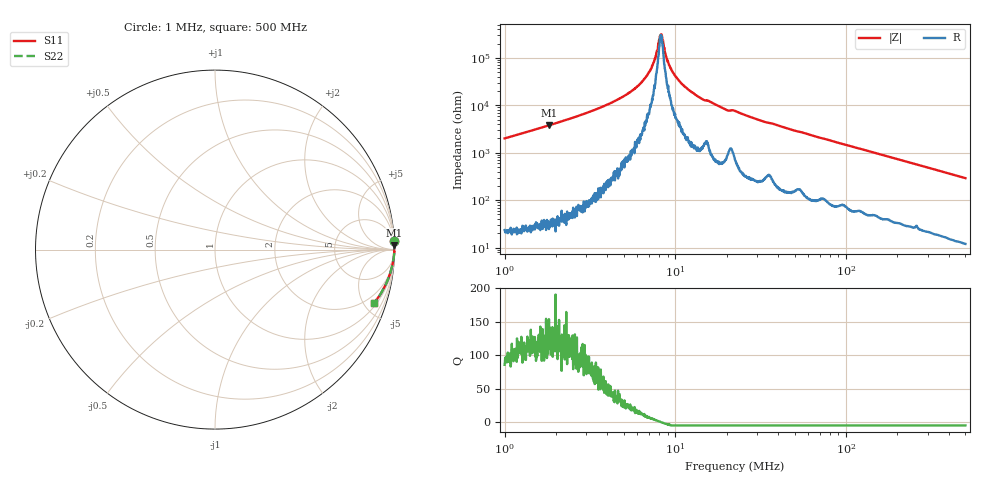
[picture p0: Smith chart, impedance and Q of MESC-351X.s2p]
!s-Parameter Generated by FASTRON Sdn. Bhd.
!FASTRON P/N : MESC-351X
!Keysight Technologies,E4991B,MY54100416,A.01.15
!Date: Fri Mar 27 11:36:06 2026
!Version  : Rev00 Fri Mar 27 11:36:06 2026
!Data & Calibration Information:
!PortZ  Port1:50+j0  Port2:50+j0
!When reading, reference impedance value at option line is always used.
!Remarks : This data is being provided solely for informational purposes.
!Freq	S11	S21	S12	S22
# Hz S dB R 50
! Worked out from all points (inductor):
!   1601 points, 1 MHz to 500 MHz, reference 50 ohm
!   read as one part in series: L = 315 uH near 1.032 MHz
!   highest Q = 132 at 1.819 MHz (marker M1), where L = 331 uH
!   self-resonance near 8.209 MHz
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1000000  -0.02 2.9  -26.06 -86.5  -26.06 -86.5  -0.02 2.9
1818762  -0.00 1.5  -31.56 -88.1  -31.56 -88.1  -0.00 1.5
2820919  -0.00 0.9  -36.02 -88.5  -36.02 -88.5  -0.00 0.9
4392302  -0.00 0.5  -41.70 -87.8  -41.70 -87.8  -0.00 0.5
6016274  -0.00 0.2  -48.07 -85.9  -48.07 -85.9  -0.00 0.2
6629778  -0.00 0.2  -51.37 -83.0  -51.37 -83.0  -0.00 0.2
7165329  -0.00 0.1  -55.05 -80.4  -55.05 -80.4  -0.00 0.1
7654427  -0.00 0.1  -60.62 -71.9  -60.62 -71.9  -0.00 0.1
7957584  -0.00 0.0  -66.06 -57.5  -66.06 -57.5  -0.00 0.0
8176910  -0.00 0.0  -69.60 -16.1  -69.60 -16.1  -0.00 0.0
8337263  -0.00 -0.0  -69.68 22.9  -69.68 22.9  -0.00 -0.0
8941017  -0.00 -0.1  -59.11 72.5  -59.11 72.5  -0.00 -0.1
9404074  -0.00 -0.1  -55.57 77.7  -55.57 77.7  -0.00 -0.1
1.020329e7  -0.00 -0.2  -51.55 82.3  -51.55 82.3  -0.00 -0.2
1.141981e7  -0.00 -0.2  -47.70 84.5  -47.70 84.5  -0.00 -0.2
1.447295e7  -0.01 -0.4  -42.52 84.1  -42.52 84.1  -0.01 -0.4
1.997865e7  -0.01 -0.7  -38.02 83.5  -38.02 83.5  -0.01 -0.7
2.236068e7  -0.01 -0.7  -37.65 83.9  -37.65 83.9  -0.01 -0.7
3.310225e7  -0.01 -1.3  -33.09 85.3  -33.09 85.3  -0.01 -1.3
6.307767e7  -0.02 -2.5  -27.35 85.2  -27.35 85.2  -0.02 -2.5
1.77937e8  -0.11 -6.8  -18.47 80.5  -18.47 80.5  -0.11 -6.8
5e8  -0.59 -18.7  -9.89 69.0  -9.89 69.0  -0.59 -18.7
